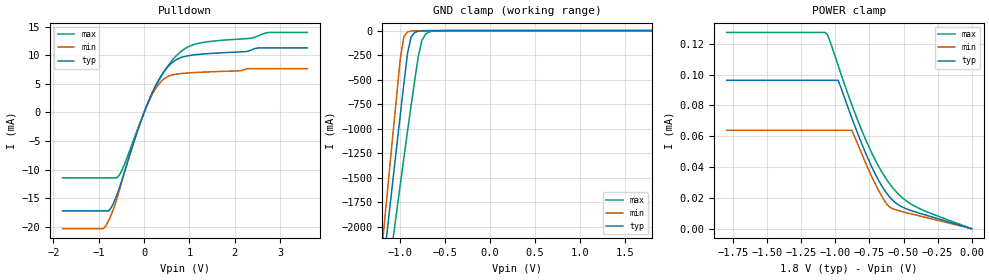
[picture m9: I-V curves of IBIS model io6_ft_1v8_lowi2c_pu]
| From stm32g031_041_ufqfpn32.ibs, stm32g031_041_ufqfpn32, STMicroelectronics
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[Model]  io6_ft_1v8_lowi2c_pu
Model_type I/O_open_drain
Polarity   Non-Inverting
Enable   Active-Low
Vinl =   0.540000V
Vinh =   1.260000V
Vmeas =  0.900000V
Cref =   40.000000pF
Rref =   100.000000M
Vref =   0.0V
C_comp   1.277600pF   1.236700pF   1.315100pF
[Temperature Range]   25.000000   -40.000000   0.125000k
[Pullup Reference]   1.800000V   1.600000V   2.000000V
[Pulldown Reference]   0.0V   0.0V   0.0V
[POWER Clamp Reference]   1.800000V   1.600000V   2.000000V
[GND Clamp Reference]   0.0V   0.0V   0.0V
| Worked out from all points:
|   slope of the pulldown table from 0 to 0.27 V, typ, clamps not added: 54.7 ohm
|   GND clamp passes 1 mA (typ) near -0.66 V on its own axis
[Pulldown]
|Voltage   I(typ)   I(min)   I(max)
-1.8V     -17.22mA   -20.33mA   -11.45mA
-900mV    -17.22mA   -20.33mA   -11.45mA
-720mV    -16.58mA   -17.82mA   -11.45mA
-600mV    -14.41mA   -15.08mA   -11.45mA
-480mV    -11.58mA   -11.79mA   -9.954mA
0V        0A         0A         0A
240mV     4.49mA     3.999mA    4.291mA
480mV     7.563mA    6.085mA    7.612mA
780mV     9.487mA    6.76mA     10.43mA
1.14V     10.08mA    6.976mA    11.96mA
2.76V     11.26mA    7.647mA    13.98mA
3.6V      11.26mA    7.647mA    13.98mA
[GND_clamp]
|Voltage   I(typ)   I(min)   I(max)
-1.8V     -7.471A    -7.973A    -7.298A
-1.2V     -2.489A    -2.18A     -2.954A
-1.16V    -2.16A     -1.797A    -2.674A
-1.08V    -1.505A    -1.034A    -2.118A
-1V       -857.9mA   -283.1mA   -1.568A
-960mV    -540.4mA   -62.14mA   -1.296A
-920mV    -234.4mA   -13.75mA   -1.028A
-880mV    -66.29mA   -4.855mA   -765.3mA
-800mV    -6.505mA   -2.056mA   -266mA
-760mV    -3.074mA   -1.45mA    -100.4mA
-680mV    -1.215mA   -557.1uA   -14.19mA
1.8V      0A         0A         0A
[POWER_clamp]
|Voltage   I(typ)   I(min)   I(max)
-1.8V     96.34uA    63.94uA    127.5uA
-1.08V    96.34uA    63.94uA    127.5uA
-1.06V    96.34uA    63.94uA    126.3uA
-980mV    96.34uA    63.94uA    105.8uA
-880mV    71.93uA    63.94uA    80.41uA
-800mV    53.62uA    47.15uA    62.36uA
-720mV    37.64uA    31.24uA    46.77uA
-640mV    25.08uA    18.16uA    34.09uA
-600mV    20.4uA     13.93uA    28.92uA
-520mV    14.54uA    11.31uA    20.97uA
-420mV    11.06uA    9.102uA    14.71uA
0V        0A         0A         0A
[Ramp]
| variable   typ   min   max
dV/dt_r  0.306/98.29899n   0.210/95.43765n   0.369/0.11291u
dV/dt_f  0.29976/96.98901n   0.21210/0.10064u   0.36510/96.17500n
R_load = 50.000000
